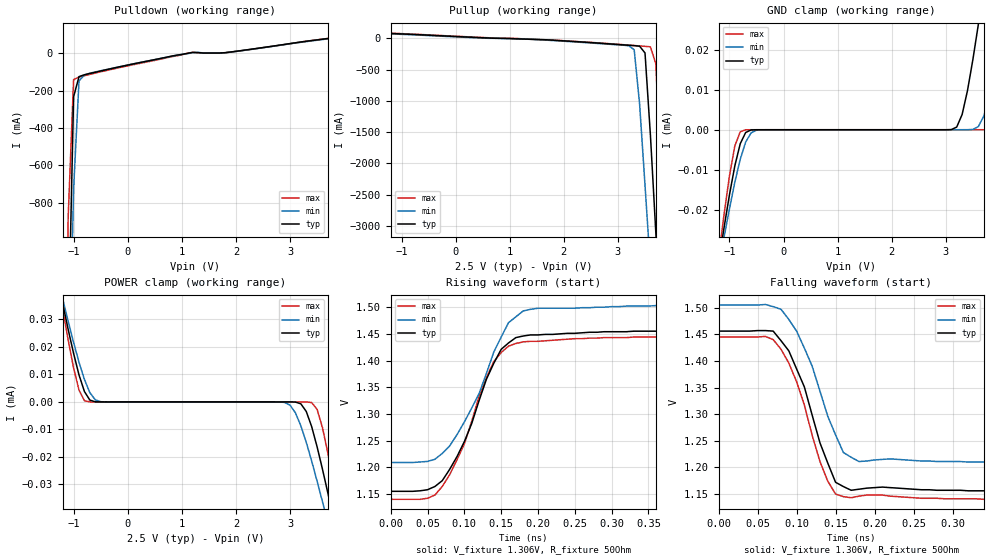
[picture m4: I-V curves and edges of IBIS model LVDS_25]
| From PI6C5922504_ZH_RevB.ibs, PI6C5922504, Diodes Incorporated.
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| Model  OUTPUT LVDS_25
[Model]  LVDS_25
Model_type  Output
Vmeas =   1.31
|Variable   typ   min   max
C_comp   1.93p   1.91p  1.96p
|Variable   typ   min   max
[Voltage Range]   2.5   2.375   2.625
[Temperature Range]   25   85   -40
[Pullup Reference]   2.5   2.375   2.625
[Pulldown Reference]   0   0   0
[Power Clamp Reference]   2.5   2.375   2.625
[GND Clamp Reference]   0   0   0
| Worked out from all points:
|   slope of the pulldown table from 0 to 0.375 V, typ, clamps not added: 17.1 ohm
|   slope of the pullup table from 0 to 0.375 V, typ, clamps not added: 24.7 ohm
|   falling waveform, V_fixture 1.306V, R_fixture 50Ohm: 20-80 % time 41.3ps typ, 44.8ps min, 39.3ps max; typ from 1.46 V to 1.16 V
|   rising waveform, V_fixture 1.306V, R_fixture 50Ohm: 20-80 % time 52.3ps typ, 57.7ps min, 50ps max; typ from 1.16 V to 1.46 V
[GND Clamp]
| Voltage   I(typ)   I(min)  I(max)
-2.5V     -159uA     -141uA     -188uA
-1.2V     -33.2uA    -34.4uA    -31.9uA
-1.1V     -24.5uA    -26.9uA    -21.2uA
-900mV    -9uA       -13.1uA    -4.02uA
-700mV    -692nA     -3.07uA    -12.5nA
3.2V      664nA      15.6pA     5.6pA
3.6V      26.3uA     787nA      7.2pA
4.1V      75.3uA     29.3uA     9.75pA
4.4V      106uA      54.1uA     451nA
4.5V      117uA      62.6uA     4.28uA
4.7V      138uA      80.1uA     22.5uA
5V        170uA      107uA      57.4uA
[POWER Clamp]
| Voltage   I(typ)   I(min)  I(max)
-2.5V     170uA      152uA      197uA
-1.3V     45.2uA     45.6uA     45.3uA
-1.2V     35.6uA     37.3uA     33.6uA
-1V       17.6uA     21.6uA     12.3uA
-800mV    3.79uA     8.18uA     451nA
-500mV    983pA      78.9nA     7.8pA
2.9V      -37.3pA    -183nA     -6.35pA
3.1V      -51nA      -3.97uA    -7.34pA
3.4V      -9uA       -21.5uA    -239nA
3.6V      -24.5uA    -36.3uA    -9.41uA
3.9V      -51.5uA    -60uA      -40.2uA
5V        -159uA     -152uA     -173uA
[Pulldown]
| Voltage   I(typ)   I(min)  I(max)
-2.5V     -23.4A     -20.3A     -28.9A
-1.2V     -3.11A     -3.33A     -2.87A
-1.1V     -1.55A     -2.03A     -874mA
-1V       -233mA     -726mA     -141mA
-900mV    -125mA     -148mA     -127mA
-800mV    -115mA     -116mA     -120mA
-700mV    -108mA     -107mA     -113mA
1V        -6.52mA    -6.42mA    -8.61mA
1.2V      4.47mA     2.55mA     4.77mA
1.7V      1.09mA     1.07mA     1.04mA
1.9V      6.45mA     5.66mA     5.86mA
5V        126mA      125mA      126mA
[Pullup]   |Note: Vtable = Vcc - Voutput
| Voltage   I(typ)   I(min)  I(max)
-2.5V     126mA      120mA      131mA
500mV     10.2mA     4.79mA     14.5mA
1.4V      -14.4mA    -14.8mA    -14.5mA
3.2V      -110mA     -118mA     -107mA
3.3V      -116mA     -181mA     -114mA
3.4V      -125mA     -1.05A     -121mA
3.5V      -233mA     -2.35A     -127mA
3.6V      -1.55A     -3.66A     -135mA
3.7V      -3.11A     -4.96A     -405mA
3.8V      -4.68A     -6.26A     -2.37A
3.9V      -6.24A     -7.56A     -4.37A
5V        -23.4A     -21.9A     -26.4A
[Falling Waveform]
V_fixture = 1.306V
V_fixture_min = 1.357V
V_fixture_max = 1.292V
R_fixture = 50Ohm
C_fixture = 0F
|   Time   V(typ)   V(min)   V(max)
0s        1.456V     1.505V     1.445V
60ps      1.457V     1.506V     1.446V
80ps      1.438V     1.497V     1.422V
110ps     1.351V     1.424V     1.317V
130ps     1.246V     1.343V     1.211V
140ps     1.208V     1.296V     1.174V
150ps     1.172V     1.261V     1.15V
160ps     1.164V     1.228V     1.145V
180ps     1.159V     1.211V     1.146V
980ps     1.155V     1.209V     1.14V
[Rising Waveform]
V_fixture = 1.306V
V_fixture_min = 1.357V
V_fixture_max = 1.292V
R_fixture = 50Ohm
C_fixture = 0F
|   Time   V(typ)   V(min)   V(max)
0s        1.155V     1.209V     1.14V
50ps      1.158V     1.211V     1.142V
70ps      1.175V     1.226V     1.164V
100ps     1.248V     1.285V     1.244V
120ps     1.325V     1.338V     1.333V
140ps     1.395V     1.416V     1.398V
170ps     1.443V     1.482V     1.432V
200ps     1.448V     1.498V     1.436V
320ps     1.454V     1.502V     1.443V
980ps     1.456V     1.505V     1.445V
[Ramp]
|   typ   min   max
dV/dt_r   0.1801/51.51E-12   0.1769/65.45E-12   0.1826/49.60E-12
dV/dt_f   0.1801/41.22E-12   0.1769/48.99E-12   0.1826/39.24E-12
R_load =   50.0000
